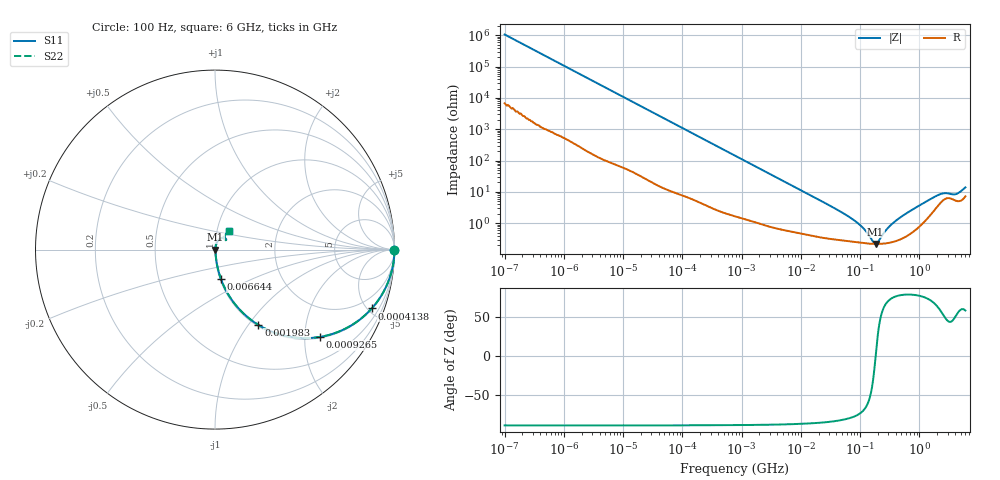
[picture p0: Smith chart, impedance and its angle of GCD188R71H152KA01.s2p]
!Murata Part Number: GCD188R71H152KA01
!These Parameters are Measured in Series Mode Connection
!Data Generated on Jan 08, 2026
!  o--ll--o
!Port1  Port2
!  o------o
!Operation Temp=25[degC], DC Bias Voltage=0[V]
!Freq. Start=100[Hz] Stop=6[GHz] 401[Steps]
# Hz S RI R 50
!Freq.(Hz) S11(Real) S11(Imag) S21(Real) S21(Imag) S12(Real) S12(Imag) S22(Real) S22(Imag)
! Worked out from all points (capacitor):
!   401 points, 100 Hz to 6 GHz, reference 50 ohm
!   read as one part in series: C = 1.49 nF near 109 Hz
!   lowest |Z| = 217 mohm at 182.6 MHz (marker M1)
!   series resonance near 183.3 MHz, so ESL is about 510 pH
!   S11 on the Smith chart (normalised r, x): 100 Hz: open; 413.8 kHz: 1.05, -5.31; 926.5 kHz: 1.03, -2.38; 1.983 MHz: 1.02, -1.12; 6.644 MHz: 1.01, -0.34; 6 GHz: 1.14, +0.24
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100  1 -9.36e-05  6e-07 9.36e-05  6e-07 9.36e-05  1 -9.36e-05
2008  1 -0.00186  1.21e-05 0.00186  1.21e-05 0.00186  1 -0.00186
40335  0.9984 -0.037  0.00158 0.037  0.00158 0.037  0.9984 -0.037
147774  0.9811 -0.1324  0.0189 0.1324  0.0189 0.1324  0.9811 -0.1324
413847  0.8736 -0.3278  0.1264 0.3278  0.1264 0.3278  0.8736 -0.3278
774597  0.6676 -0.4653  0.3324 0.4653  0.3324 0.4653  0.6676 -0.4653
926525  0.5855 -0.4864  0.4145 0.4864  0.4145 0.4864  0.5855 -0.4864
1983483  0.2423 -0.4199  0.7577 0.4199  0.7577 0.4199  0.2423 -0.4199
3394479  0.1025 -0.2925  0.8975 0.2925  0.8975 0.2925  0.1025 -0.2925
6644369  0.0326 -0.1623  0.9674 0.1623  0.9674 0.1623  0.0326 -0.1623
1.555665e7  0.00907 -0.0716  0.9909 0.0716  0.9909 0.0716  0.00907 -0.0716
8.154455e7  0.00262 -0.0116  0.9974 0.0116  0.9974 0.0116  0.00262 -0.0116
1.166697e8  0.00233 -0.00608  0.9977 0.00608  0.9977 0.00608  0.00233 -0.00608
1.669249e8  0.00218 -0.00123  0.9978 0.00123  0.9978 0.00123  0.00218 -0.00123
1.825626e8  0.00216 -5e-05  0.9978 5e-05  0.9978 5e-05  0.00216 -5e-05
1.996653e8  0.00217 0.00114  0.9978 -0.00114  0.9978 -0.00114  0.00217 0.00114
3.124326e8  0.00241 0.00745  0.9976 -0.00745  0.9976 -0.00745  0.00241 0.00745
5.847788e8  0.004 0.0192  0.996 -0.0192  0.996 -0.0192  0.004 0.0192
1.791126e9  0.0287 0.0603  0.9713 -0.0603  0.9713 -0.0603  0.0287 0.0603
2.562649e9  0.0562 0.0641  0.9438 -0.0641  0.9438 -0.0641  0.0562 0.0641
4.193612e9  0.0531 0.061  0.9469 -0.061  0.9469 -0.061  0.0531 0.061
6e9  0.0785 0.1022  0.9215 -0.1022  0.9215 -0.1022  0.0785 0.1022
